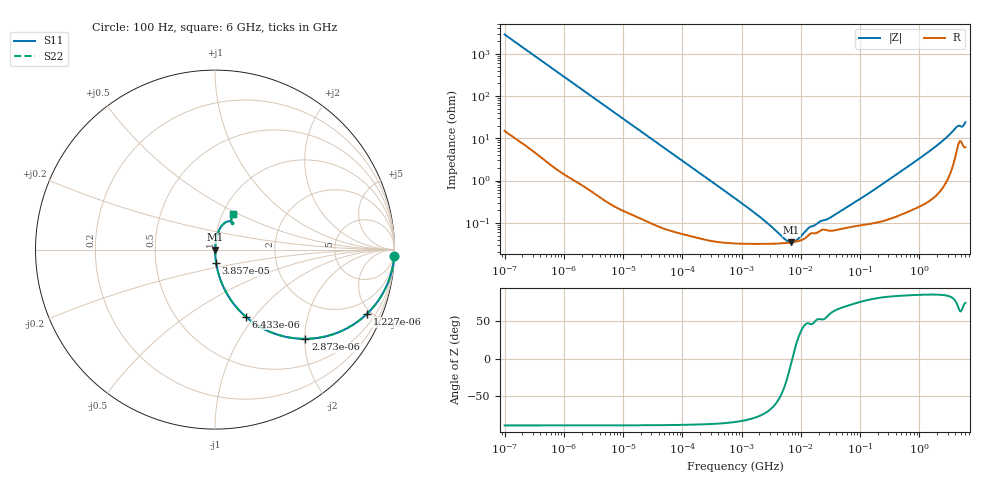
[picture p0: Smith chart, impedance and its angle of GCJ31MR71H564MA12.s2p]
!Murata Part Number: GCJ31MR71H564MA12
!These Parameters are Measured in Series Mode Connection
!Data Generated on Mar 13, 2026
!  o--ll--o
!Port1  Port2
!  o------o
!Operation Temp=25[degC], DC Bias Voltage=0[V]
!Freq. Start=100[Hz] Stop=6[GHz] 401[Steps]
# Hz S RI R 50
!Freq.(Hz) S11(Real) S11(Imag) S21(Real) S21(Imag) S12(Real) S12(Imag) S22(Real) S22(Imag)
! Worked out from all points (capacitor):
!   401 points, 100 Hz to 6 GHz, reference 50 ohm
!   read as one part in series: C = 555 nF near 109 Hz
!   lowest |Z| = 34.4 mohm at 6.949 MHz (marker M1)
!   series resonance near 7.178 MHz, so ESL is about 890 pH
!   S11 on the Smith chart (normalised r, x): 100 Hz: 1, -57; 1.227 kHz: 1.02, -4.71; 2.873 kHz: 1.01, -2.02; 6.433 kHz: 1.01, -0.90; 38.57 kHz: 1.00, -0.15; 6 GHz: 1.12, +0.47
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100  0.9986 -0.0348  0.0014 0.0348  0.0014 0.0348  0.9986 -0.0348
401  0.9803 -0.1364  0.0197 0.1364  0.0197 0.1364  0.9803 -0.1364
750  0.9356 -0.243  0.0644 0.243  0.0644 0.243  0.9356 -0.243
1227  0.8457 -0.3587  0.1543 0.3587  0.1543 0.3587  0.8457 -0.3587
2008  0.6738 -0.4661  0.3262 0.4661  0.3262 0.4661  0.6738 -0.4661
2873  0.5039 -0.4972  0.4961 0.4972  0.4961 0.4972  0.5039 -0.4972
6433  0.1706 -0.3733  0.8294 0.3733  0.8294 0.3733  0.1706 -0.3733
13169  0.0479 -0.21  0.9521 0.21  0.9521 0.21  0.0479 -0.21
38569  0.00652 -0.0752  0.9935 0.0752  0.9935 0.0752  0.00652 -0.0752
40335  0.00602 -0.072  0.994 0.072  0.994 0.072  0.00602 -0.072
774597  0.000338 -0.00378  0.9997 0.00378  0.9997 0.00378  0.000338 -0.00378
2372521  0.000318 -0.00111  0.9997 0.00111  0.9997 0.00111  0.000318 -0.00111
5554849  0.000332 -0.000215  0.9997 0.000215  0.9997 0.000215  0.000332 -0.000215
6948629  0.000343 -2.69e-05  0.9997 2.69e-05  0.9997 2.69e-05  0.000343 -2.69e-05
8692127  0.000363 0.000161  0.9996 -0.000161  0.9996 -0.000161  0.000363 0.000161
1.300572e7  0.000482 0.000528  0.9995 -0.000528  0.9995 -0.000528  0.000482 0.000528
1.555665e7  0.000571 0.000601  0.9994 -0.000601  0.9994 -0.000601  0.000571 0.000601
3.184506e7  0.000649 0.00117  0.9994 -0.00117  0.9994 -0.00117  0.000649 0.00117
3.124326e8  0.00133 0.0106  0.9987 -0.0106  0.9987 -0.0106  0.00133 0.0106
1.712697e9  0.00705 0.0568  0.993 -0.0568  0.993 -0.0568  0.00705 0.0568
4.193612e9  0.0686 0.1562  0.9314 -0.1562  0.9314 -0.1562  0.0686 0.1562
6e9  0.1012 0.1971  0.8988 -0.1971  0.8988 -0.1971  0.1012 0.1971
